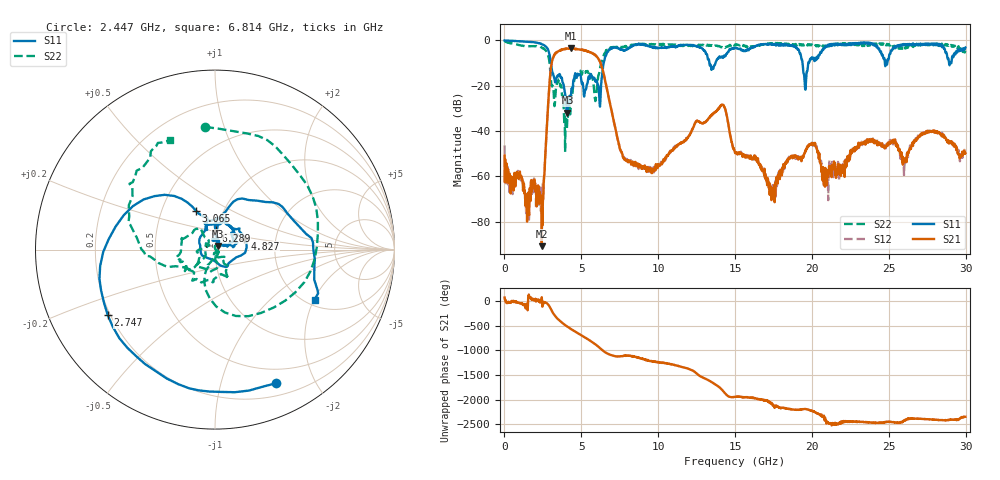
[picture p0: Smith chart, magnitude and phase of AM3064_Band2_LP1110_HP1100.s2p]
# Hz S DB R 50.0
!freq dBS11 angS11 dBS21 angS21 dBS12 angS12 dBS22 angS22
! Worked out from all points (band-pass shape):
!   1600 points, 10 MHz to 29.98 GHz, reference 50 ohm
!   highest |S21| = -3.51 dB at 4.321 GHz (marker M1); lowest = -90.9 dB at 2.428 GHz (marker M2)
!   |S21| within 3 dB of the highest: 3.23 GHz to 5.908 GHz (2.678 GHz wide, 58.6 % of centre)
!   lowest |S11| = -32.0 dB at 4.096 GHz (marker M3), VSWR 1.05, Z = 51.4 + j2.11 ohm
!   |S11| at or under -10 dB: 3.02 GHz to 6.45 GHz (3.43 GHz wide, 72.4 % of centre); 13.33 GHz to 13.72 GHz (390.5 MHz wide, 2.89 % of centre); 19.39 GHz to 19.76 GHz (371.8 MHz wide, 1.9 % of centre)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
!   |S22| runs from -49.2 to -0.2 dB; largest |S21 - S12| = 0.021
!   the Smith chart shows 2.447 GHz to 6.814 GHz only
!   S11 on the Smith chart (normalised r, x): 2.447 GHz: 0.33, -1.51; 2.747 GHz: 0.19, -0.27; 3.065 GHz: 0.74, +0.34; 4.827 GHz: 1.38, +0.17; 6.289 GHz: 0.98, +0.21; 6.814 GHz: 2.23, -2.02
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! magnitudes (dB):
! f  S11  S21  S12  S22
! 10 MHz  0.0  -50.8  -46.3  -0.2
! 1.472 GHz  -0.6  -80.0  -72.1  -2.6
! 2.428 GHz  -1.7  -90.9  -74.0  -3.1
! 2.447 GHz  -1.7  -74.1  -77.8  -3.3
! 2.747 GHz  -3.1  -39.5  -39.3  -5.1
! 3.065 GHz  -12.3  -10.1  -10.1  -20.1
! 4.096 GHz  -32.0  -3.6  -3.6  -33.7
! 4.321 GHz  -24.9  -3.5  -3.6  -27.8
! 4.827 GHz  -15.1  -3.9  -3.9  -14.4
! 5.015 GHz  -18.4  -4.1  -4.1  -15.3
! 5.914 GHz  -18.0  -6.6  -6.6  -26.8
! 6.289 GHz  -19.4  -10.8  -10.7  -10.2
! 6.814 GHz  -4.1  -26.4  -26.4  -3.6
! 7.826 GHz  -4.5  -52.1  -52.5  -2.7
! 10 GHz  -3.3  -55.9  -55.2  -1.8
! 14.14 GHz  -7.3  -28.6  -28.5  -2.9
! 15 GHz  -3.2  -49.7  -49.3  -2.0
! 17.46 GHz  -1.5  -66.2  -68.8  -1.3
! 19.99 GHz  -7.5  -45.5  -45.8  -1.8
! 20.95 GHz  -2.8  -62.0  -57.8  -2.2
! 25 GHz  -8.1  -45.3  -45.8  -1.6
! 29.98 GHz  -3.1  -49.7  -47.9  -4.6
